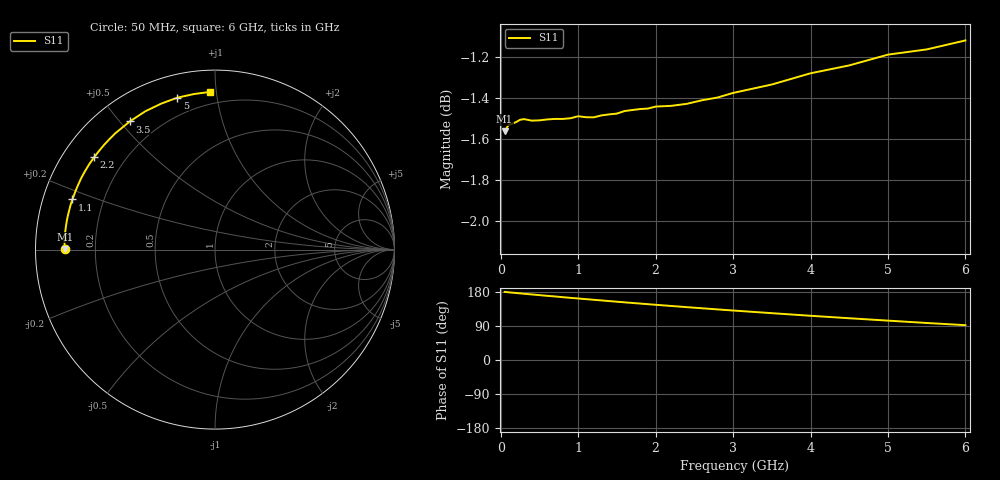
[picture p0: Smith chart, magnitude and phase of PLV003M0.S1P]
! Infineon Technologies  Discrete & RF Semiconductors
! BAR 64-04W /-05W /-06W
! Si PIN Diode in SOT323
! IF = 3 mA
! S-Parameters:  October  2008
# GHz  S  MA  R  50
!  f  S11
! GHz  MAG  ANG
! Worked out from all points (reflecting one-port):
!   34 points, 50 MHz to 6 GHz, reference 50 ohm
!   lowest |S11| = -1.6 dB at 50 MHz (marker M1), VSWR 11.15, Z = 4.48 + j0.0866 ohm
!   phase of S11 starts at 180 deg and turns -88 deg over the sweep
!   S11 on the Smith chart (normalised r, x): 50 MHz: 0.09, +0.00; 1.1 GHz: 0.09, +0.17; 2.2 GHz: 0.09, +0.34; 3.5 GHz: 0.10, +0.53; 5 GHz: 0.11, +0.78; 6 GHz: 0.12, +0.96
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0.05  0.8355 179.8
0.1  0.8383 178.7
0.2  0.8397 176.7
0.25  0.8408 175.8
0.3  0.8411 174.8
0.6  0.8409 169.4
0.7  0.8412 167.6
0.8  0.8412 165.8
0.9  0.8415 164.0
1  0.8424 162.3
1.1  0.842 160.6
1.3  0.8428 157.2
1.5  0.8437 153.8
1.6  0.8449 152.2
1.7  0.8454 150.5
1.8  0.8458 148.9
2  0.847 145.7
2.2  0.8474 142.6
2.4  0.8483 139.5
2.6  0.85 136.5
2.8  0.8513 133.5
3  0.8535 130.6
3.5  0.8575 123.6
4  0.8629 116.7
4.5  0.8668 110.2
5  0.872 103.9
5.5  0.8745 97.7
6  0.8789 91.9
